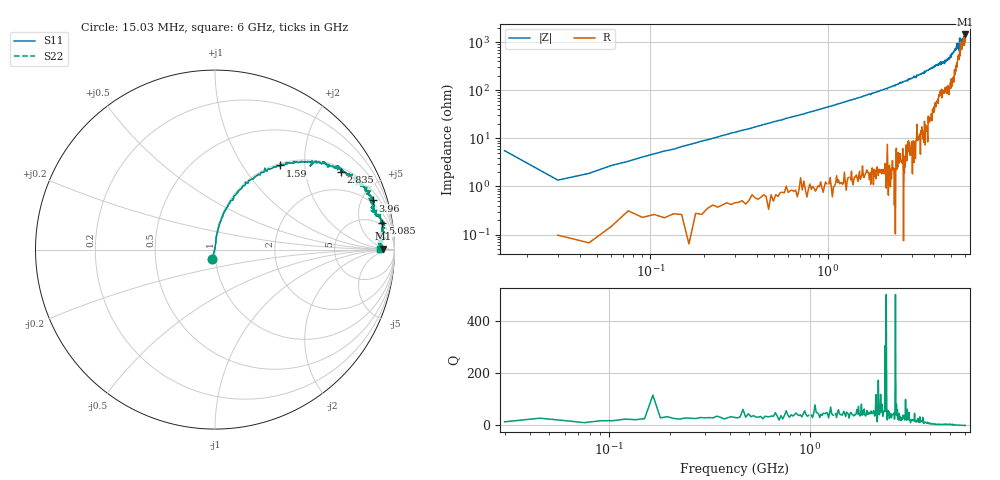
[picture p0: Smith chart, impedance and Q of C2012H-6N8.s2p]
!	Network	Analyzer	HP8753E.07.74:	Oct	30	2002	Serial	No.	JP38451487
!	Hewlett-Packard
!	28	Aug	2009	9:39:59
!	Frequency	S11	S21	S12	S22
#	HZ	S	RI	R	50
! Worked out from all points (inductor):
!   400 points, 15.03 MHz to 6 GHz, reference 50 ohm
!   read as one part in series: L = 7.07 nH near 45.03 MHz
!   highest |Z| = 1.44 kohm at 5.985 GHz (marker M1)
!   self-resonance near 5.954 GHz
!   S11 on the Smith chart (normalised r, x): 15.03 MHz: 0.96, -0.10; 1.59 GHz: 1.04, +1.50; 2.835 GHz: 1.17, +3.15; 3.96 GHz: 1.71, +6.09; 5.085 GHz: 4, +11; 6 GHz: 24, +2
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1.502992e7  -0.0156 -0.0537  1.02 0.0537  1.02 0.0537  -0.0156 -0.0537
3.002985e7  0.00131 0.0135  0.999 -0.0135  0.999 -0.0135  0.00131 0.0135
1.200294e8  0.00536 0.0541  0.995 -0.0541  0.995 -0.0541  0.00536 0.0541
2.850286e8  0.0203 0.125  0.98 -0.125  0.98 -0.125  0.0203 0.125
1.020025e9  0.179 0.371  0.821 -0.371  0.821 -0.371  0.179 0.371
1.590022e9  0.362 0.469  0.638 -0.469  0.638 -0.469  0.362 0.469
2.01002e9  0.498 0.489  0.502 -0.489  0.502 -0.489  0.498 0.489
2.835016e9  0.703 0.431  0.297 -0.431  0.297 -0.431  0.703 0.431
3.015015e9  0.765 0.419  0.235 -0.419  0.235 -0.419  0.765 0.419
3.96001e9  0.878 0.274  0.122 -0.274  0.122 -0.274  0.878 0.274
4.00501e9  0.888 0.265  0.112 -0.265  0.112 -0.265  0.888 0.265
5.010005e9  0.932 0.158  0.0684 -0.158  0.0684 -0.158  0.932 0.158
5.085005e9  0.933 0.148  0.0667 -0.148  0.0667 -0.148  0.933 0.148
5.355003e9  0.952 0.0907  0.0484 -0.0907  0.0484 -0.0907  0.952 0.0907
5.535002e9  0.902 0.0932  0.0978 -0.0932  0.0978 -0.0932  0.902 0.0932
5.565002e9  0.95 0.0612  0.0496 -0.0612  0.0496 -0.0612  0.95 0.0612
5.595002e9  0.91 0.0811  0.0896 -0.0811  0.0896 -0.0811  0.91 0.0811
5.625002e9  0.934 0.0398  0.0661 -0.0398  0.0661 -0.0398  0.934 0.0398
5.865001e9  0.933 0.0213  0.0669 -0.0213  0.0669 -0.0213  0.933 0.0213
5.925e9  0.913 0.0388  0.0866 -0.0388  0.0866 -0.0388  0.913 0.0388
5.985e9  0.935 0.00549  0.0646 -0.00549  0.0646 -0.00549  0.935 0.00549
6e9  0.919 0.0058  0.0813 -0.0058  0.0813 -0.0058  0.919 0.0058
